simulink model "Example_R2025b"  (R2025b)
settings: Solver=VariableStepAuto  StartTime=0.0  StopTime=100  RelTol=1e-3
libraries: MotionSystems_Simulink_R2025b x2

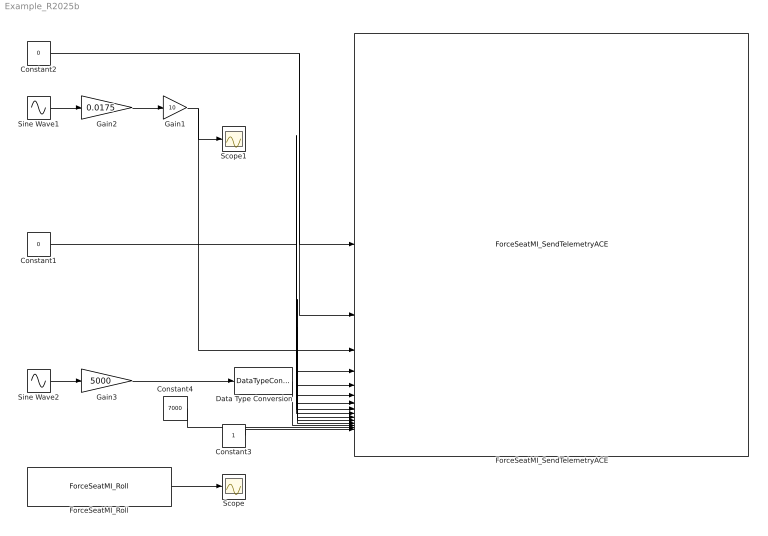
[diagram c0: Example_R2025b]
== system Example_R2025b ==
  Constant1 : Constant  Value=0  OutDataTypeStr=double
  Constant2 : Constant  Value=0
  Constant3 : Constant  OutDataTypeStr=int32
  Constant4 : Constant  Value=7000  OutDataTypeStr=int32
  Data Type Conversion : DataTypeConversion
  ForceSeatMI_Roll : MotionSystems_Simulink_R2025b/ForceSeatMI_Roll  SampleTime=-1
  ForceSeatMI_SendTelemetryACE : MotionSystems_Simulink_R2025b/ForceSeatMI_SendTelemetryACE  SampleTime=-1
  Gain1 : Gain  Gain=10
  Gain2 : Gain  Gain=0.0175
  Gain3 : Gain  Gain=5000
  Scope : Scope
  Scope1 : Scope
  Sine Wave1 : Sin  SampleTime=0.01
  Sine Wave2 : Sin  SampleTime=0.01
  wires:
  Constant1/1 -> ForceSeatMI_SendTelemetryACE/12, ForceSeatMI_SendTelemetryACE/11, ForceSeatMI_SendTelemetryACE/10, ForceSeatMI_SendTelemetryACE/9, ForceSeatMI_SendTelemetryACE/8, ForceSeatMI_SendTelemetryACE/7, ForceSeatMI_SendTelemetryACE/6, ForceSeatMI_SendTelemetryACE/5, ForceSeatMI_SendTelemetryACE/4
  Constant2/1 -> ForceSeatMI_SendTelemetryACE/2, ForceSeatMI_SendTelemetryACE/1
  Sine Wave1/1 -> Gain2/1
  Gain2/1 -> Gain1/1
  Gain1/1 -> ForceSeatMI_SendTelemetryACE/3, Scope1/1
  ForceSeatMI_Roll/1 -> Scope/1
  Constant3/1 -> ForceSeatMI_SendTelemetryACE/15
  Constant4/1 -> ForceSeatMI_SendTelemetryACE/14
  Sine Wave2/1 -> Gain3/1
  Gain3/1 -> Data Type Conversion/1
  Data Type Conversion/1 -> ForceSeatMI_SendTelemetryACE/13
